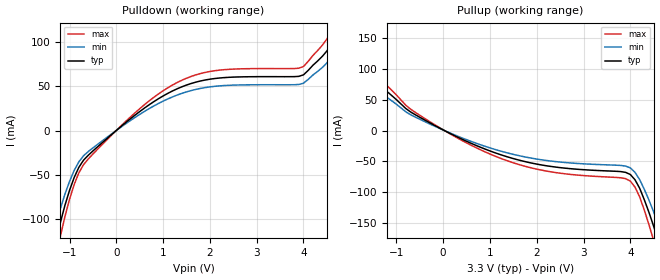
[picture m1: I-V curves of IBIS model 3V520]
[IBIS Ver]   2.1
[File name]   574_3.ibs
[File Rev]   2.0
[Date]   06/12/01
[Source]   ICS MicroClock Applications Engineering 2
[Disclaimer] This information is for modeling purposes only, and is
(C) Copyright Integrated Circuit Systems, Inc. 1997-2001
   All rights reserved
ICS hereby grants the user of this IBIS model a non-exclusive,
nontransferable license to use this IBIS model under the following terms.
Before using this IBIS model, the user should read this license.
If the user does not accept these terms,  the IBIS model should be
returned to ICS within 30 days.
   The user is granted this license only to use the IBIS model and
is not granted rights to sell, load, rent, lease or license the IBIS
model in whole or in part, or in modified form to anyone other than
user. User may modify the IBIS model to suit its specific
applications but rights to derivative works and such modifications
shall belong to ICS.
   This IBIS model is provided on an "AS IS" basis and ICS makes
absolutely no warranty with respect to the information contained
herein. ICS DISCLAIMS AND CUSTOMER WAIVES ALL WARRANTIES, EXPRESS
OR IMPLIED, INCLUDING WARRANTIES OF MERCHANTABILITY OR FITNESS FOR
A PARTICULAR PURPOSE. The entire risk as to quality and performance
is with the Customer. ACCORDINGLY, IN NO EVENT SHALL THE COMPANY BE
LIABLE FOR ANY DAMAGES, WHETHER IN CONTRACT OR TORT,INCLUDING ANY
LOST PROFITS OR OTHER INCIDENTAL, CONSEQUENTIAL, EXEMPLARY, OR
PUNITIVE DAMAGES ARISING OUT OF THE USE OR APPLICATION OF THE IBIS
model provided in this package. Further, ICS reserves the right to
make changes without notice to any product herein to improve
reliability, function, or design. ICS does not convey any license
under patent rights or any other intellectual property rights,
including those of third parties.
   ICS is not obligated to provide maintenance or support
for the licensed IBIS model.
[Component]   ICS574
[Manufacturer] Integrated Circuit Systems Inc.
[Package]
|   typ   min   max
R_pkg   40m   35m   45m
L_pkg   1.65nH   1.35nH   1.95nH
C_pkg   0.24pF   0.14pF   0.34pF
[pin]   signal_name   model_name   R_pin   L_pin   C_pin
   2   CLK1   3V520
   3   CLK2   3V520
   6   CLK3   3V520
   7   CLK4   3V520
| Models and submodels in the file (1): 3V520 (Output)
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|   ICS754 3.3V Clock Drive Model
| This model is suitable for all output pins on the
| ICS574
[Model]   3V520
Model_type   Output
Polarity   Non-Inverting
|   typ   min   max
C_comp   5pF   4pF   6pF
|   typ   min   max
[Voltage range]  3.3V   3.15V   3.45V
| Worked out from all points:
|   slope of the pulldown table from 0 to 0.495 V, typ, clamps not added: 23.4 ohm
|   slope of the pullup table from 0 to 0.495 V, typ, clamps not added: 27 ohm
[pulldown]
|Voltage I (typ)   I (min)   I (max)
-3.3V     -3A        -3A        -3A
-1.4V     -147mA     -125mA     -169.1mA
-1.2V     -104.7mA   -88.98mA   -120.4mA
-900mV    -52.9mA    -44.96mA   -60.83mA
-700mV    -33.44mA   -28.43mA   -38.46mA
500mV     21.37mA    18.16mA    24.57mA
1.4V      49.25mA    41.86mA    56.64mA
4V        62.74mA    53.33mA    72.15mA
4.5V      89.6mA     76.16mA    103mA
4.7V      111.9mA    95.14mA    128.7mA
4.9V      150mA      127.5mA    172.5mA
6.6V      3A         3A         3A
[pullup]
|Voltage I (typ)   I (min)   I (max)
-3.3V     3A         3A         3A
-2.2V     178.3mA    151.5mA    205mA
-2.1V     158.9mA    135mA      182.7mA
-1.8V     109.5mA    93.05mA    125.9mA
-1.4V     76.99mA    65.45mA    88.54mA
-700mV    30.37mA    25.82mA    34.93mA
200mV     -6.72mA    -5.71mA    -7.73mA
1.8V      -51.44mA   -43.72mA   -59.15mA
4V        -71.53mA   -60.8mA    -82.26mA
4.5V      -156.2mA   -132.8mA   -179.6mA
4.7V      -199.9mA   -169.9mA   -229.9mA
6.6V      -3A        -3A        -3A
[Ramp]
|   typ   min   max
dV/dt_r   1.26/0.45n   1.19/0.49n   1.32/0.40n
dV/dt_f   1.33/0.42n   1.26/0.46n   1.40/0.37n
